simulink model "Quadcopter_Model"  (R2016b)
settings: Solver=VariableStepAuto  StartTime=0.0  StopTime=10.0  RelTol=1e-3
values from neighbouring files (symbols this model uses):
  If = 0.511    [modelParameters.m]    (also in thrustDragConstantCalculations.m = [If0; If1; If2; If3]; Kd_error.m = I_0 * sign(rotor_speed_0) + I_1 * rotor_speed_0 + I_2 * roto)
  Jreq = 4.2012e-05    [modelParameters.m]
  Jxx = 0.0218    [modelParameters.m]
  Jyy = 0.0277    [modelParameters.m]
  Jzz = 0.0332    [modelParameters.m]
  Kd = 1.8087e-07    [modelParameters.m]    (also in calcDragConstant.m = ((A'*A)^-1)*A'*b; thrustDragConstantCalculations.m = calcDragConstant(data, Pmin, Pmax, Rm, Kv, Kq, If ))
  Kq = 96.3422    [modelParameters.m]    (also in thrustDragConstantCalculations.m; Kd_error.m)
  Kt = 8.1558*10^-6    (= 8.1558e-06)    [modelParameters.m]    (also in calcThrustConstant.m = ((A'*A)^(-1))*(A'*T); thrustDragConstantCalculations.m = calcThrustConstant(data))
  Kv = 96.3422    [modelParameters.m]    (also in thrustDragConstantCalculations.m; Kd_error.m)
  m = 1.19    [modelParameters.m]
  Pmax = 0.80    (= 0.8)    [modelParameters.m]    (also in thrustDragConstantCalculations.m; Kd_error.m)
  Pmin = 0.47    [modelParameters.m]    (also in thrustDragConstantCalculations.m = 0.4; Kd_error.m = 0.4)
  rhx = 0.016    [modelParameters.m]
  rhy = 0.016    [modelParameters.m]
  rhz = 0.003    [modelParameters.m]
  Rm = 0.2308    [modelParameters.m]    (also in thrustDragConstantCalculations.m; Kd_error.m)
  Vb = 11.1    [modelParameters.m]    (also in calcDragConstant.m = [data.(6); data.(6); data.(6); data.(6)]; Kd_error.m = data.(6))

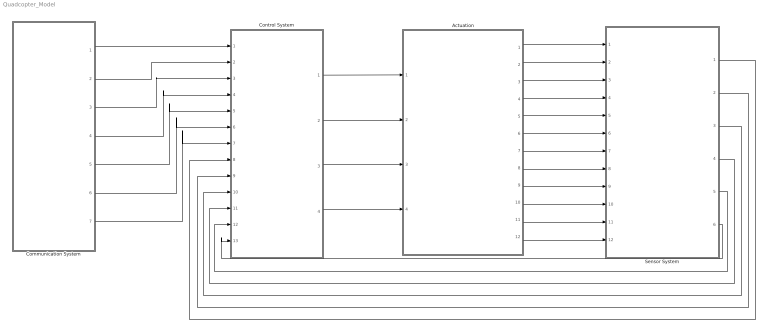
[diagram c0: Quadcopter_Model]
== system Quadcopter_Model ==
  Actuation : Subsystem
  Communication System : Subsystem
  Control System : Subsystem
  Sensor System : Subsystem
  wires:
  Control System/1(Rotor 0 Duty Cycle) -> Actuation/1(Rotor 0 Duty Cycle)
  Control System/2(Rotor 1 Duty Cycle) -> Actuation/2(Rotor 1 Duty Cycle)
  Actuation/4(Body frame angular velocity (p)) -> Sensor System/4(Body frame angular velocity (p))
  Actuation/5(Body frame angular velocity (q)) -> Sensor System/5(Body frame angular velocity (q))
  Actuation/6(Body frame angular velocity (r)) -> Sensor System/6(Body frame angular velocity (r))
  Sensor System/6(Yaw rate (psi dot)) -> Control System/13(Yaw rate (psi dot))
  Sensor System/5(Roll rate (theta dot)) -> Control System/12(Roll rate (theta dot))
  Sensor System/4(Pitch rate (phi dot)) -> Control System/11(Pitch rate (phi dot))
  Sensor System/3(Yaw (psi)) -> Control System/10(Yaw (psi))
  Sensor System/2(Roll (theta)) -> Control System/9(Roll (theta))
  Sensor System/1(Pitch (phi)) -> Control System/8(Pitch (phi))
  Communication System/1(x_position) -> Control System/1(x position)
  Communication System/2(y_position) -> Control System/2(y position)
  Communication System/3(z_position) -> Control System/3(z position)
  Communication System/4(x_setpoint) -> Control System/4(x setpoint)
  Communication System/5(y_setpoint) -> Control System/5(y setpoint)
  Communication System/6(z_setpoint) -> Control System/6(z setpoint)
  Communication System/7(yaw_setpoint) -> Control System/7("Yaw setpoint ")
  Control System/3(Rotor 2 Duty Cycle) -> Actuation/3(Rotor 2 Duty Cycle)
  Control System/4(Rotor 3 Duty Cycle) -> Actuation/4(Rotor 3 Duty Cycle)
  Actuation/7(Earth frame position (x)) -> Sensor System/7(Earth frame position (x))
  Actuation/8(Earth frame position (y)) -> Sensor System/8(Earth frame position (y))
  Actuation/9(Earth frame position (z)) -> Sensor System/9(Earth frame position (z))
  Actuation/10(Earth frame pitch (phi)) -> Sensor System/10(Earth frame pitch (phi))
  Actuation/11(Earth frame roll (theta)) -> Sensor System/11(Earth frame roll (theta))
  Actuation/12(Earth frame yaw (psi)) -> Sensor System/12(Earth frame yaw (psi))
  Actuation/1(Body frame linear velocity (u)) -> Sensor System/1(Body frame linear velocity (u))
  Actuation/2(Body frame linear velocity (v)) -> Sensor System/2(Body frame linear velocity (v))
  Actuation/3(Body frame linear velocity (w)) -> Sensor System/3(Body frame linear velocity (w))

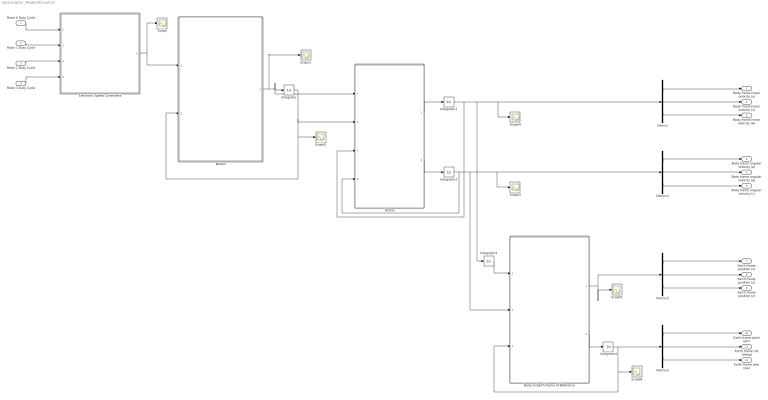
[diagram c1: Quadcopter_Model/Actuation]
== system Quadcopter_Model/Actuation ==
  Rotor 0 Duty Cycle : Inport
  Rotor 1 Duty Cycle : Inport  Port=2
  Rotor 2 Duty Cycle : Inport  Port=3
  Rotor 3 Duty Cycle : Inport  Port=4
  Body to Earth Frame of Reference : MATLAB Function  TreatAsAtomicUnit=on
  Demux{,1..3} (4 alike) : Demux  Outputs=3
  Electronic Speed Controllers : MATLAB Function  TreatAsAtomicUnit=on
  Integrator{,1..4} (5 alike) : Integrator
  Motors : MATLAB Function  TreatAsAtomicUnit=on
  Rotors : MATLAB Function  TreatAsAtomicUnit=on
  Scope{,1..6} (7 alike) : Scope
  Body frame linear velocity (u) : Outport
  Body frame linear velocity (v) : Outport  Port=2
  Body frame linear velocity (w) : Outport  Port=3
  Body frame angular velocity (p) : Outport  Port=4
  Body frame angular velocity (q) : Outport  Port=5
  Body frame angular velocity (r) : Outport  Port=6
  Earth frame position (x) : Outport  Port=7
  Earth frame position (y) : Outport  Port=8
  Earth frame position (z) : Outport  Port=9
  Earth frame pitch (phi) : Outport  Port=10
  Earth frame roll (theta) : Outport  Port=11
  Earth frame yaw (psi) : Outport  Port=12
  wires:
  Rotor 3 Duty Cycle/1 -> Electronic Speed Controllers/4(rotor_3_duty_cycle)
  Rotor 2 Duty Cycle/1 -> Electronic Speed Controllers/3(rotor_2_duty_cycle)
  Rotor 1 Duty Cycle/1 -> Electronic Speed Controllers/2(rotor_1_duty_cycle)
  Rotor 0 Duty Cycle/1 -> Electronic Speed Controllers/1(rotor_0_duty_cycle)
  Electronic Speed Controllers/1(Vb_eff) -> Scope/1, Motors/1(Vb_eff)
  Motors/1(angular_acceleration) -> Scope1/1, Rotors/1(angular_acceleration), Integrator/1
  Integrator/1 -> Rotors/2(angular_velocity), Scope2/1, Motors/2(angular_velocity)
  Rotors/2(bOmega_dot) -> Integrator2/1
  Rotors/1(b_v_dot) -> Integrator1/1
  Integrator2/1 -> Body to Earth Frame of Reference/2(bOmega), Demux1/1, Scope3/1, Rotors/4(bOmega)
  Integrator1/1 -> Rotors/3(b_v), Integrator3/1, Demux/1, Scope4/1
  Demux/1 -> Body frame linear velocity (u)/1
  Demux/2 -> Body frame linear velocity (v)/1
  Demux/3 -> Body frame linear velocity (w)/1
  Demux1/1 -> Body frame angular velocity (p)/1
  Demux1/3 -> Body frame angular velocity (r)/1
  Demux1/2 -> Body frame angular velocity (q)/1
  Integrator3/1 -> Body to Earth Frame of Reference/1(body_frame_position)
  Body to Earth Frame of Reference/2(euler_rates) -> Integrator4/1
  Demux3/1 -> Earth frame pitch (phi)/1
  Demux3/2 -> Earth frame roll (theta)/1
  Demux3/3 -> Earth frame yaw (psi)/1
  Demux2/3 -> Earth frame position (z)/1
  Demux2/2 -> Earth frame position (y)/1
  Demux2/1 -> Earth frame position (x)/1
  Integrator4/1 -> Scope6/1, Body to Earth Frame of Reference/3(euler_angles), Demux3/1
  Body to Earth Frame of Reference/1(earth_frame_position) -> Demux2/1, Scope5/1

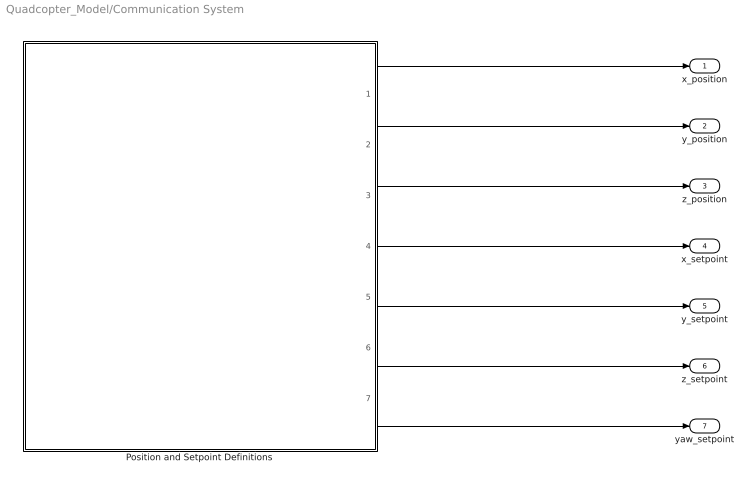
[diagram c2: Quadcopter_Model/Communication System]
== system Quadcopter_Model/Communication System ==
  Position and Setpoint Definitions : MATLAB Function  TreatAsAtomicUnit=on
  x_position : Outport
  y_position : Outport  Port=2
  z_position : Outport  Port=3
  x_setpoint : Outport  Port=4
  y_setpoint : Outport  Port=5
  z_setpoint : Outport  Port=6
  yaw_setpoint : Outport  Port=7
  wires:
  Position and Setpoint Definitions/7(yaw_setpoint) -> yaw_setpoint/1
  Position and Setpoint Definitions/6(z_setpoint) -> z_setpoint/1
  Position and Setpoint Definitions/5(y_setpoint) -> y_setpoint/1
  Position and Setpoint Definitions/4(x_setpoint) -> x_setpoint/1
  Position and Setpoint Definitions/3(z_position) -> z_position/1
  Position and Setpoint Definitions/2(y_position) -> y_position/1
  Position and Setpoint Definitions/1(x_position) -> x_position/1

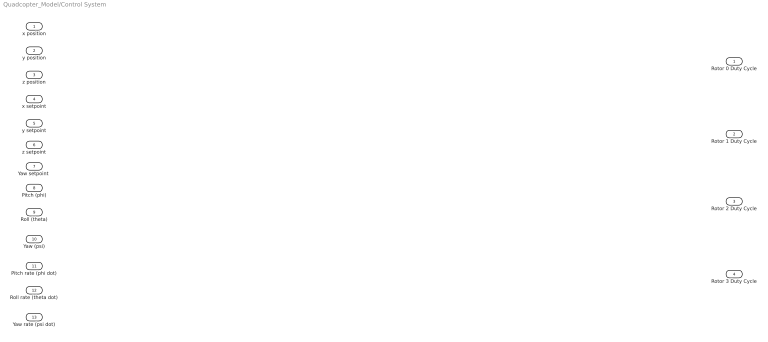
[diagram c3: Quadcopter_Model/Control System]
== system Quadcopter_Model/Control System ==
  x position : Inport
  y position : Inport  Port=2
  z position : Inport  Port=3
  x setpoint : Inport  Port=4
  y setpoint : Inport  Port=5
  z setpoint : Inport  Port=6
  "Yaw setpoint " : Inport  Port=7
  Pitch (phi) : Inport  Port=8
  Roll (theta) : Inport  Port=9
  Yaw (psi) : Inport  Port=10
  Pitch rate (phi dot) : Inport  Port=11
  Roll rate (theta dot) : Inport  Port=12
  Yaw rate (psi dot) : Inport  Port=13
  Rotor 0 Duty Cycle : Outport
  Rotor 1 Duty Cycle : Outport  Port=2
  Rotor 2 Duty Cycle : Outport  Port=3
  Rotor 3 Duty Cycle : Outport  Port=4

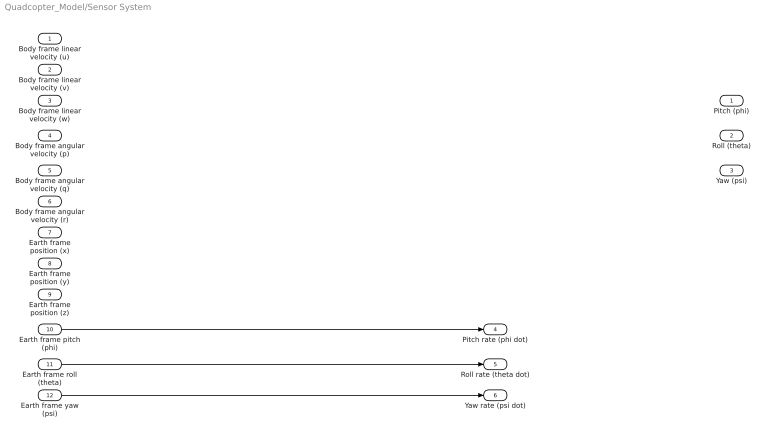
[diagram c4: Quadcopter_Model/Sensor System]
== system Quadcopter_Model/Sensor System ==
  Body frame linear velocity (u) : Inport
  Body frame linear velocity (v) : Inport  Port=2
  Body frame linear velocity (w) : Inport  Port=3
  Body frame angular velocity (p) : Inport  Port=4
  Body frame angular velocity (q) : Inport  Port=5
  Body frame angular velocity (r) : Inport  Port=6
  Earth frame position (x) : Inport  Port=7
  Earth frame position (y) : Inport  Port=8
  Earth frame position (z) : Inport  Port=9
  Earth frame pitch (phi) : Inport  Port=10
  Earth frame roll (theta) : Inport  Port=11
  Earth frame yaw (psi) : Inport  Port=12
  Pitch (phi) : Outport
  Roll (theta) : Outport  Port=2
  Yaw (psi) : Outport  Port=3
  Pitch rate (phi dot) : Outport  Port=4
  Roll rate (theta dot) : Outport  Port=5
  Yaw rate (psi dot) : Outport  Port=6
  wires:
  Earth frame pitch (phi)/1 -> Pitch rate (phi dot)/1
  Earth frame roll (theta)/1 -> Roll rate (theta dot)/1
  Earth frame yaw (psi)/1 -> Yaw rate (psi dot)/1

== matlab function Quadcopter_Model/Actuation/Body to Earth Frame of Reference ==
function [earth_frame_position, euler_rates] = body_earth_conversion(body_frame_position, bOmega, euler_angles)

euler_rates = zeros(3,1);
earth_frame_position = zeros(3,1);

phi = euler_angles(1);
theta = euler_angles(2);
psi = euler_angles(3);

Aeb = [1, sin(phi)*tan(theta), cos(phi)*tan(theta); ...
       0,     cos(phi)       ,        -sin(phi)   ; ...
       0  sin(phi)/cos(theta), cos(phi)/cos(theta);];

Leb = [cos(theta)*cos(psi), sin(phi)*sin(theta)*cos(psi)-cos(phi)*sin(psi), cos(phi)*sin(theta)*cos(psi)+sin(phi)*sin(psi); ...
       cos(theta)*cos(psi), sin(phi)*sin(theta)*cos(psi)+cos(phi)*sin(psi), cos(phi)*sin(theta)*cos(psi)-sin(phi)*sin(psi); ...
           -sin(theta)    ,                sin(phi)*cos(theta)            ,                 cos(phi)*cos(theta)           ;];

euler_rates = Aeb * bOmega;

earth_frame_position = Leb * body_frame_position;

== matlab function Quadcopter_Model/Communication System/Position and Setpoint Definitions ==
function [x_position, y_position, z_position, x_setpoint,...
    y_setpoint, z_setpoint, yaw_setpoint]= positionAndSetpointDefinitions

x_position = 0;
y_position = 0;
z_position = 0;
x_setpoint = 0;
y_setpoint = 0;
z_setpoint = 0;
yaw_setpoint = 0;

end

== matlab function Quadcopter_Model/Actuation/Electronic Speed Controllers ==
function Vb_eff   = ESC(rotor_0_duty_cycle, rotor_1_duty_cycle, rotor_2_duty_cycle, rotor_3_duty_cycle, Pmin, Pmax, Vb)

% Define u_Pi for each of the rotors
u_P0 = (rotor_0_duty_cycle/100 - Pmin) / (Pmax - Pmin);
u_P1 = (rotor_1_duty_cycle/100 - Pmin) / (Pmax - Pmin);
u_P2 = (rotor_2_duty_cycle/100 - Pmin) / (Pmax - Pmin);
u_P3 = (rotor_3_duty_cycle/100 - Pmin) / (Pmax - Pmin);

% Determine the effective battery voltage from each ESC
Vb_eff_0 = u_P0 * Vb;
Vb_eff_1 = u_P1 * Vb;
Vb_eff_2 = u_P2 * Vb;
Vb_eff_3 = u_P3 * Vb;

Vb_eff = [Vb_eff_0, Vb_eff_1, Vb_eff_2, Vb_eff_3];

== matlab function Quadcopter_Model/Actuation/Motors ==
function angular_acceleration  = motor(Vb_eff, angular_velocity, Rm, Kv, Kq, Kd, If, Jreq)

angular_acceleration = zeros(1,4);

% Define each motors effective battery voltage
Vb_eff_0 = Vb_eff(1);
Vb_eff_1 = Vb_eff(2);
Vb_eff_2 = Vb_eff(3);
Vb_eff_3 = Vb_eff(4);

% Determine the angular velocity of each rotor from feedback
w_0 = angular_velocity(1);
w_1 = angular_velocity(2);
w_2 = angular_velocity(3);
w_3 = angular_velocity(4);

% Determine angular acceleration of each rotor
w_0_dot = 1/(Jreq*Rm*Kq) * Vb_eff_0 - 1/(Jreq*Rm*Kq*Kv) * w_0 - 1/(Jreq*Kq)*If - (Kd/Jreq) * w_0^2;
w_1_dot = 1/(Jreq*Rm*Kq) * Vb_eff_1 - 1/(Jreq*Rm*Kq*Kv) * w_1 - 1/(Jreq*Kq)*If - (Kd/Jreq) * w_1^2;
w_2_dot = 1/(Jreq*Rm*Kq) * Vb_eff_2 - 1/(Jreq*Rm*Kq*Kv) * w_2 - 1/(Jreq*Kq)*If - (Kd/Jreq) * w_2^2;
w_3_dot = 1/(Jreq*Rm*Kq) * Vb_eff_3 - 1/(Jreq*Rm*Kq*Kv) * w_3 - 1/(Jreq*Kq)*If - (Kd/Jreq) * w_3^2;

angular_acceleration = [w_0_dot, w_1_dot, w_2_dot, w_3_dot];

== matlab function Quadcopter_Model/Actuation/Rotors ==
function [b_v_dot, bOmega_dot]= rotor(angular_acceleration, angular_velocity, b_v, bOmega, m, Kt, Kd, rhx, rhy, rhz, Jreq, Jxx, Jyy, Jzz)

b_v_dot = zeros(3,1);
bOmega_dot = zeros(3,1);

% Create J vector
J = [Jxx,  0 ,  0 ; ...
      0 , Jyy,  0 ; ...
      0 ,  0 , Jzz;];

% Create r_hi vector
rh_0 = [-rhx; -rhy; rhz];
rh_1 = [-rhx; rhy; rhz];
rh_2 = [rhx; -rhy; rhz];
rh_3 = [rhx; rhy; rhz];

% Define vector from body frame origin to center of mass
br_oc = [0; 0; 0];

% Define 3x3 Identity Matrix
I = eye(3);

% Create gamma vectors
gamma_Ti = [0; 0; -1];
gamma_omega_03 = [0; 0; -1];  %Rotors 0 and 3 use this gamma_omega vector
gamma_omega_12 = [0; 0; 1]; %Rotors 1 and 2 use this gamma_omega vector

% Define angular velocities for each rotor
w_0 = angular_velocity(1);
w_1 = angular_velocity(2);
w_2 = angular_velocity(3);
w_3 = angular_velocity(4);

% Define angular acceleration for each rotor
w_0_dot = angular_acceleration(1);
w_1_dot = angular_acceleration(2);
w_2_dot = angular_acceleration(3);
w_3_dot = angular_acceleration(4);

% Define the body force in the z-direction from each rotor
bF_0 = Kt * w_0 * w_0 * gamma_Ti;
bF_1 = Kt * w_1 * w_1 * gamma_Ti;
bF_2 = Kt * w_2 * w_2 * gamma_Ti;
bF_3 = Kt * w_3 * w_3 * gamma_Ti;

% Sum up the body forces in the z-direction from each vector to get the
% total body force in the z-direction
bF = bF_0 + bF_1 + bF_2 + bF_3;

% Define the in-plane drag and induced torque produced by each rotor
 bQ_d0 = -1 * Kd * w_0 * w_0 * gamma_omega_03;
 bQ_d1 = -1 * Kd * w_1 * w_1 * gamma_omega_12;
 bQ_d2 = -1 * Kd * w_2 * w_2 * gamma_omega_12;
 bQ_d3 = -1 * Kd * w_3 * w_3 * gamma_omega_03;

% Sum up the total in-plane drag and induced torque to get the total
% in-plane drag and induced torque on the body
bQ_d = bQ_d0 + bQ_d1 + bQ_d2 + bQ_d3;

% Define the force lever arm torque created from the force produced by each
% rotor in the z-direction
bQ_F0 = cross( rh_0, bF_0 );
bQ_F1 = cross( rh_1, bF_1 );
bQ_F2 = cross( rh_2, bF_2 );
bQ_F3 = cross( rh_3, bF_3 );

bQ_F = bQ_F0 + bQ_F1 + bQ_F2 + bQ_F3;

%Define the change in angular momentum torque produced by each rotor 
bQ_L0 = -1 * Jreq * ( cross(bOmega, w_0 * gamma_omega_03) + w_0_dot * gamma_omega_03 );
bQ_L1 = -1 * Jreq * ( cross(bOmega, w_1 * gamma_omega_12) + w_1_dot * gamma_omega_12 ); 
bQ_L2 = -1 * Jreq * ( cross(bOmega, w_2 * gamma_omega_12) + w_2_dot * gamma_omega_12 ); 
bQ_L3 = -1 * Jreq * ( cross(bOmega, w_3 * gamma_omega_03) + w_3_dot * gamma_omega_03 );

% Sum up the total change in angular momentum torque produced by each rotor
bQ_L = bQ_L0 + bQ_L1 + bQ_L2 + bQ_L3;

% Define the total rotor system torque as the sum of the in-plane drag and
% induced torque, force lever arm torque, and change in angular momentum
% torques
bQ = bQ_d + bQ_F + bQ_L;

% Define the body frame linear velocities
b_v_dot = (m*I)^(-1) * ( bF - cross( bOmega, m*(b_v + cross(bOmega, br_oc)) ) );

% Define the body frame angular velocities
bOmega_dot = J ^(-1) * ( bQ - cross(bOmega, J * bOmega) - cross(br_oc, bF) );
